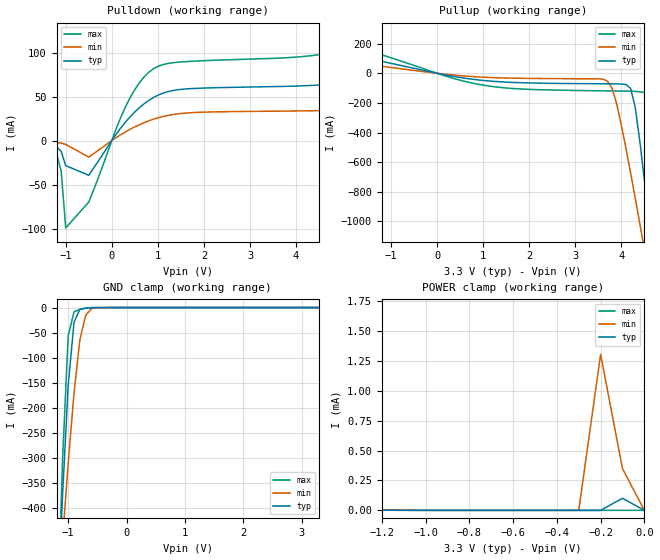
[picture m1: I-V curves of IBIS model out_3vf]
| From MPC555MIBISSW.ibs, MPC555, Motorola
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|   OUTPUT_3VF(50pf load)
[Model]   out_3vf
Model_type   Output
Polarity   Non-Inverting
|   typ   min   max
C_comp   6.7080e-13   6.0050e-13   7.6470e-13
| CAP models
| typical : model= typ
| maximum : model= wcs
| minimum : model= bcs
[Voltage range]   3.3v   3.0v   3.6v
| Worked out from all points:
|   slope of the pulldown table from 0 to 0.495 V, typ, clamps not added: 15.3 ohm
|   slope of the pullup table from 0 to 0.495 V, typ, clamps not added: 17.5 ohm
|   GND clamp passes 1 mA (typ) near -0.70 V on its own axis
|   POWER clamp passes 1 mA (typ) near -2.50 V on its own axis
|  typical: model = typ,  temp = 25,  vdd = 3.3
|  maximum: model = bcs,  temp = -40, vdd = 3.6
|  minimum: model = wcs,  temp = 150, vdd = 3.0
[Pulldown]
|  Voltage   I(typ)   I(min)   I(max)
-9V       -57.85mA   -7.714mA   -109.7mA
-6V       -46.97mA   -21.95mA   -82.43mA
-3.3V     -830uA     -300uA     -1.4mA
-1.3V     -4.911mA   -1.631mA   -8.96mA
-1.1V     -12.31mA   -2.871mA   -34.49mA
-1V       -28.48mA   -4.35mA    -99.26mA
-500mV    -39.47mA   -18.79mA   -69.93mA
300mV     21.25mA    10.05mA    38.67mA
900mV     48.81mA    24.2mA     81.5mA
5.6V      71.39mA    38.01mA    114mA
6.1V      164.9mA    151mA      195.5mA
6.6V      416.3mA    321.6mA    530.3mA
[GND_clamp]
-3.3V     -6.942A    -4.403A    -10.42A
-1.2V     -648.1mA   -632.8mA   -705.4mA
-1.1V     -383mA     -468.1mA   -313.1mA
-1V       -154.9mA   -311.4mA   -56.14mA
-900mV    -29.19mA   -170.4mA   -8.377mA
-800mV    -3.643mA   -64.63mA   -3.772mA
-700mV    -1.021mA   -15.21mA   -1.258mA
-600mV    -239.5uA   -2.066mA   -170.3uA
-400mV    -1.896uA   -47.44uA   -129.1nA
3.3V      52.74pA    15.4nA     1.967nA
[Pullup]
-3.3V     209.8mA    131.3mA    298.5mA
900mV     -45.04mA   -24.66mA   -74.38mA
3.6V      -71.02mA   -39.58mA   -118.5mA
3.8V      -71.46mA   -102.4mA   -119.2mA
4.1V      -75.67mA   -506.1mA   -120.3mA
4.3V      -227.5mA   -840.4mA   -122.3mA
4.4V      -455.7mA   -1.013A    -125.1mA
4.6V      -1.001A    -1.364A    -178.6mA
4.7V      -1.288A    -1.541A    -436mA
4.8V      -1.581A    -1.719A    -828.5mA
4.9V      -1.876A    -1.899A    -1.258A
6.6V      -7.027A    -4.996A    -9.158A
[POWER_clamp]
-3.3V     326.4mA    252.4mA    344.4mA
-2.9V     131.9mA    17.75mA    208.9mA
-2.7V     43.4mA     113.1uA    142.8mA
-2.6V     10.66mA    99.3uA     110.6mA
-2.4V     64.47uA    81.32uA    49.87mA
-2.2V     36.14uA    64.17uA    6.272mA
-2V       27.04uA    47.68uA    93.46uA
-1.9V     22.74uA    39.53uA    18.75uA
-300mV    62.04pA    51.07nA    15.43nA
-200mV    65.85pA    1.303mA    15.55nA
-100mV    101uA      348.4uA    16.09nA
0V        45.46pA    40.86pA    12.46nA
| RAMP models
| typical dv/dt : model=typ, temp=25
| maximum dv/dt : model=bcs, temp=-40
| minimum dv/dt : model=wcs, temp=150
|		 typ   min   max
[Ramp]
dV/dt_r	 1.52577/3.23061E-10   0.941414/3.884E-10   2.25156/1.85321E-10
dV/dt_f  1.52577/3.02278E-10   0.941414/4.27607E-10   2.25156/1.73518E-10
